|   Microchip Technology Inc.
|   RT-PolarFire IBIS Model
[IBIS ver]   5.0
[File name]   rt-polarfire_hsio_se.ibs
[File Rev]   1.3
[Date]   Thu June 05 2025
[Source] Simulated Models ONLY.
   All data is based on Spice simulation. All performed at Microchip Technology Inc.
[Notes]   This IBIS file is for HSIO single ended standards.
   Please refer to rt-polarfire_hsio_diff.ibs for HSIO differential Standards Configurations,
   and refer to rt-polarfire_gpio_se.ibs and rt-polarfire_gpio_diff.ibs for GPIO Configurations.
   The package parasitics of various package types are given.
   Uncomment the appropriate package before simulations.
   Revision History
   Rev 1.3: 05-Jun-2025
   - Added RLC information for RTPF500ZT-FCG1509 Die-Package combination
   - Added RLC information for RTPF500ZT-CG1509 Die-Package combination
   - Added RLC information for RTPF500ZT-LG1509 Die-Package combination
   - Added RLC information for RTPF500T-LG1509 Die-Package combination
   - This IBIS model file is applicable to all RTPF500T variants
   - RTPF500T/TL/TLS/TS
   - RTPF500ZT/ZTL/ZTLS/ZTS
   Rev 1.2: 22-Nov-2023
   - Added mixed mode receiver support:
   - Input buffers: LVCMOS12_135_ODT-OFF,LVCMOS12_135_ODT-120,LVCMOS12_135_ODT-240,
   HSTL12_18_ODT-OFF,HSTL12_15_ODT-OFF,HSTL12_135_ODT-OFF,
   HSTL135_18_ODT-OFF,HSTL135_15_ODT-OFF,HSTL15_18_ODT-OFF,
   HSUL12_18_ODT-OFF,HSUL12_18_ODT-60,HSUL12_18_ODT-120,HSUL12_18_ODT-240,
   HSUL12_15_ODT-OFF,HSUL12_15_ODT-60,HSUL12_15_ODT-120,HSUL12_15_ODT-240,
   HSUL12_135_ODT-OFF,HSUL12_135_ODT-60,HSUL12_135_ODT-120,HSUL12_135_ODT-240,
   POD12_18_ODT-OFF,POD12_15_ODT-OFF,POD12_135_ODT-OFF,SSTL135_18_ODT-OFF,
   SSTL135_15_ODT-OFF,SSTL15_18_ODT-OFF
   - Updated Pin and Pin Mapping section
   Rev 1.1: 6-Jul-2022
   - Added LPDDR4 LVSTL11 I/O standard
[Disclaimer] This information is for board design considerations.
   Simulation based V/I curves contained in this model file are
   considered preliminary until verified against bench
   measurements. Maximum currents may vary from part to part but
   should not exceed maximum I/V curves provided in this model file.
[Copyright]  (c) 2025, Microchip Technology Inc., All Rights Reserved.
| ADDITIONAL NOTES
| Warnings for ISSO Pullup, Pulldown currents being non-zero maybe ignored.
| The naming conventions used in the signal_name/model_name are as follows:
| SLEW-#  - Slew setting,OFF or ON represented by #
| HYST-#  - Hysteresis setting,OFF or ON represented by #
| #mA   - Driver current strength, value represented by #
| #ohm   - Driver impedance mode, value represented by #
| ODT-#   - Series on-die termination, impedance value represented by #
| C1   - Refers to Class-I driver models
| C2   - Refers to Class-II driver models
| #_I   - Refers to input models ,  model name represented by #
| #_O   - Refers to output models , model name represented by #
| IBIS MODEL CHECKLIST
| Microchip Technology Inc. is dedicated to releasing quality IBIS models to customers.
| The following items have been
| verified for this IBIS model before release:
| 1)  Checked IBIS model by the golden parser ibischk5 [Complete]
| 2)  Ensured no errors reported by golden parser
|   for the IBIS model [Complete]
| 3)  Defined Vinl and Vinh for receivers [Complete]
| 4)  Defined Standard Load and Vmeas values for drivers [Complete]
| 5)  Defined overshoots for drivers and receivers [NA]
| 6)  Validated Ramp Values[]
| 7)  Defined V-T Tables for all output drivers [Complete]
| 8)  Validated [Diff Pins] [NA]
| 9)  Verified Package Parasitics [Complete]
| 10) Defined Standard Load Parameters and Specifications
|   for waveforms [Complete]
| 11) Defined and Validate Pin mappings [Complete]
| 12) Verified C_comp_pullup and C_comp_pulldown Values []
| 13) Visually Inspected I-V Curves and V-T Tables  [Complete]
| 14) Presented Typ/Min/Max Values in the correct order for
|   all tables and parameters [Complete]
| 15) Simulated all output models with standard load and
|   switching through Vmeas [Complete]
| 16) Simulated all receiver models  [Complete]
| 17) Validated Models selectors. [NA]
| 18) Visually inspected Spice and IBIS correlation for
|   a) Typical VT Curves [Complete]
|   b) Minimum VT Curves [Complete]
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[Component]   RTPolarFire
[Manufacturer]   Microchip Technology Inc.
[Package]
|   typ   min   max
|RTPF500T
R_pkg   6.87585   NA   NA   |   RTPF500T-CG1509
L_pkg   14.5627nH   NA   NA   |   RTPF500T-CG1509
C_pkg   5.64467pF   NA   NA   |   RTPF500T-CG1509
|RTPF500T
|R_pkg   6.87585   NA   NA   |   RTPF500T-LG1509
|L_pkg   14.5627nH   NA   NA   |   RTPF500T-LG1509
|C_pkg   5.64467pF   NA   NA   |   RTPF500T-LG1509
|RTPF500ZT
|R_pkg   6.87585   NA   NA   |   RTPF500ZT-CG1509
|L_pkg   14.5627nH   NA   NA   |   RTPF500ZT-CG1509
|C_pkg   5.64467pF   NA   NA   |   RTPF500ZT-CG1509
|RTPF500ZT
|R_pkg   6.87585   NA   NA   |   RTPF500ZT-LG1509
|L_pkg   14.5627nH   NA   NA   |   RTPF500ZT-LG1509
|C_pkg   5.64467pF   NA   NA   |   RTPF500ZT-LG1509
|RTPF500ZT
|R_pkg   1.83029   NA   NA   |   RTPF500ZT-FCG1509
|L_pkg   9.9441nH   NA   NA   |   RTPF500ZT-FCG1509
|C_pkg   3.8557pF   NA   NA   |   RTPF500ZT-FCG1509
| End Header
| The PIN numbers given below are examples. They do not correspond to
| device pin numbers.
[Pin]   signal_name   model_name   R_pin   L_pin   C_pin
1   LVCMOS18_8mA_SLEW-OFF_O   LVCMOS18_8mA_SLEW-OFF_HSIO_O
2   LVCMOS18_2mA_SLEW-OFF_O   LVCMOS18_2mA_SLEW-OFF_HSIO_O
3   LVCMOS18_4mA_SLEW-OFF_O   LVCMOS18_4mA_SLEW-OFF_HSIO_O
4   LVCMOS18_6mA_SLEW-OFF_O   LVCMOS18_6mA_SLEW-OFF_HSIO_O
5   LVCMOS18_10mA_SLEW-OFF_O   LVCMOS18_10mA_SLEW-OFF_HSIO_O
6   LVCMOS18_12mA_SLEW-OFF_O   LVCMOS18_12mA_SLEW-OFF_HSIO_O
7   LVCMOS15_8mA_SLEW-OFF_O   LVCMOS15_8mA_SLEW-OFF_HSIO_O
8   LVCMOS15_2mA_SLEW-OFF_O   LVCMOS15_2mA_SLEW-OFF_HSIO_O
9   LVCMOS15_4mA_SLEW-OFF_O   LVCMOS15_4mA_SLEW-OFF_HSIO_O
10   LVCMOS15_6mA_SLEW-OFF_O   LVCMOS15_6mA_SLEW-OFF_HSIO_O
11   LVCMOS15_10mA_SLEW-OFF_O   LVCMOS15_10mA_SLEW-OFF_HSIO_O
12   LVCMOS12_8mA_SLEW-OFF_O   LVCMOS12_8mA_SLEW-OFF_HSIO_O
13   LVCMOS12_2mA_SLEW-OFF_O   LVCMOS12_2mA_SLEW-OFF_HSIO_O
14   LVCMOS12_4mA_SLEW-OFF_O   LVCMOS12_4mA_SLEW-OFF_HSIO_O
15   LVCMOS12_6mA_SLEW-OFF_O   LVCMOS12_6mA_SLEW-OFF_HSIO_O
16   LVCMOS12_10mA_SLEW-OFF_O   LVCMOS12_10mA_SLEW-OFF_HSIO_O
17   SSTL18_C1_60ohm_SLEW-OFF_O   SSTL18_C1_60ohm_SLEW-OFF_HSIO_O
18   SSTL18_C1_80ohm_SLEW-OFF_O   SSTL18_C1_80ohm_SLEW-OFF_HSIO_O
19   SSTL18_C1_48ohm_SLEW-OFF_O   SSTL18_C1_48ohm_SLEW-OFF_HSIO_O
20   SSTL18_C1_40ohm_SLEW-OFF_O   SSTL18_C1_40ohm_SLEW-OFF_HSIO_O
21   SSTL18_C2_40ohm_SLEW-OFF_O   SSTL18_C2_40ohm_SLEW-OFF_HSIO_O
22   SSTL18_C2_48ohm_SLEW-OFF_O   SSTL18_C2_48ohm_SLEW-OFF_HSIO_O
23   SSTL18_C2_34ohm_SLEW-OFF_O   SSTL18_C2_34ohm_SLEW-OFF_HSIO_O
24   SSTL18_C2_30ohm_SLEW-OFF_O   SSTL18_C2_30ohm_SLEW-OFF_HSIO_O
25   SSTL15_C1_40ohm_SLEW-OFF_O   SSTL15_C1_40ohm_SLEW-OFF_HSIO_O
26   SSTL15_C1_48ohm_SLEW-OFF_O   SSTL15_C1_48ohm_SLEW-OFF_HSIO_O
27   SSTL15_C2_34ohm_SLEW-OFF_O   SSTL15_C2_34ohm_SLEW-OFF_HSIO_O
28   SSTL15_C2_30ohm_SLEW-OFF_O   SSTL15_C2_30ohm_SLEW-OFF_HSIO_O
29   SSTL15_C2_27ohm_SLEW-OFF_O   SSTL15_C2_27ohm_SLEW-OFF_HSIO_O
30   SSTL135_C1_40ohm_SLEW-OFF_O   SSTL135_C1_40ohm_SLEW-OFF_HSIO_O
31   SSTL135_C1_48ohm_SLEW-OFF_O   SSTL135_C1_48ohm_SLEW-OFF_HSIO_O
32   SSTL135_C2_34ohm_SLEW-OFF_O   SSTL135_C2_34ohm_SLEW-OFF_HSIO_O
33   SSTL135_C2_30ohm_SLEW-OFF_O   SSTL135_C2_30ohm_SLEW-OFF_HSIO_O
34   SSTL135_C2_27ohm_SLEW-OFF_O   SSTL135_C2_27ohm_SLEW-OFF_HSIO_O
35   HSUL18_C1_55ohm_SLEW-OFF_O   HSUL18_C1_55ohm_SLEW-OFF_HSIO_O
36   HSUL18_C1_60ohm_SLEW-OFF_O   HSUL18_C1_60ohm_SLEW-OFF_HSIO_O
37   HSUL18_C1_40ohm_SLEW-OFF_O   HSUL18_C1_40ohm_SLEW-OFF_HSIO_O
38   HSUL18_C1_34ohm_SLEW-OFF_O   HSUL18_C1_34ohm_SLEW-OFF_HSIO_O
39   HSUL18_C2_25ohm_SLEW-OFF_O   HSUL18_C2_25ohm_SLEW-OFF_HSIO_O
40   HSUL18_C2_30ohm_SLEW-OFF_O   HSUL18_C2_30ohm_SLEW-OFF_HSIO_O
41   HSUL18_C2_27ohm_SLEW-OFF_O   HSUL18_C2_27ohm_SLEW-OFF_HSIO_O
42   HSUL18_C2_22ohm_SLEW-OFF_O   HSUL18_C2_22ohm_SLEW-OFF_HSIO_O
43   HSTL15_C1_50ohm_SLEW-OFF_O   HSTL15_C1_50ohm_SLEW-OFF_HSIO_O
44   HSTL15_C1_60ohm_SLEW-OFF_O   HSTL15_C1_60ohm_SLEW-OFF_HSIO_O
45   HSTL15_C1_40ohm_SLEW-OFF_O   HSTL15_C1_40ohm_SLEW-OFF_HSIO_O
46   HSTL15_C1_34ohm_SLEW-OFF_O   HSTL15_C1_34ohm_SLEW-OFF_HSIO_O
47   HSTL15_C2_25ohm_SLEW-OFF_O   HSTL15_C2_25ohm_SLEW-OFF_HSIO_O
48   HSTL15_C2_30ohm_SLEW-OFF_O   HSTL15_C2_30ohm_SLEW-OFF_HSIO_O
49   HSTL15_C2_27ohm_SLEW-OFF_O   HSTL15_C2_27ohm_SLEW-OFF_HSIO_O
50   HSTL15_C2_22ohm_SLEW-OFF_O   HSTL15_C2_22ohm_SLEW-OFF_HSIO_O
51   HSTL135_C1_50ohm_SLEW-OFF_O   HSTL135_C1_50ohm_SLEW-OFF_HSIO_O
52   HSTL135_C1_60ohm_SLEW-OFF_O   HSTL135_C1_60ohm_SLEW-OFF_HSIO_O
53   HSTL135_C1_40ohm_SLEW-OFF_O   HSTL135_C1_40ohm_SLEW-OFF_HSIO_O
54   HSTL135_C1_34ohm_SLEW-OFF_O   HSTL135_C1_34ohm_SLEW-OFF_HSIO_O
55   HSTL135_C2_25ohm_SLEW-OFF_O   HSTL135_C2_25ohm_SLEW-OFF_HSIO_O
56   HSTL135_C2_30ohm_SLEW-OFF_O   HSTL135_C2_30ohm_SLEW-OFF_HSIO_O
57   HSTL135_C2_27ohm_SLEW-OFF_O   HSTL135_C2_27ohm_SLEW-OFF_HSIO_O
58   HSTL135_C2_22ohm_SLEW-OFF_O   HSTL135_C2_22ohm_SLEW-OFF_HSIO_O
59   HSUL12_40ohm_SLEW-OFF_O   HSUL12_40ohm_SLEW-OFF_HSIO_O
60   HSUL12_120ohm_SLEW-OFF_O   HSUL12_120ohm_SLEW-OFF_HSIO_O
61   HSUL12_80ohm_SLEW-OFF_O   HSUL12_80ohm_SLEW-OFF_HSIO_O
62   HSUL12_60ohm_SLEW-OFF_O   HSUL12_60ohm_SLEW-OFF_HSIO_O
63   HSUL12_48ohm_SLEW-OFF_O   HSUL12_48ohm_SLEW-OFF_HSIO_O
64   HSUL12_34ohm_SLEW-OFF_O   HSUL12_34ohm_SLEW-OFF_HSIO_O
65   POD12_C1_48ohm_SLEW-OFF_O   POD12_C1_48ohm_SLEW-OFF_HSIO_O
66   POD12_C1_60ohm_SLEW-OFF_O   POD12_C1_60ohm_SLEW-OFF_HSIO_O
67   POD12_C1_40ohm_SLEW-OFF_O   POD12_C1_40ohm_SLEW-OFF_HSIO_O
68   POD12_C2_34ohm_SLEW-OFF_O   POD12_C2_34ohm_SLEW-OFF_HSIO_O
69   POD12_C2_30ohm_SLEW-OFF_O   POD12_C2_30ohm_SLEW-OFF_HSIO_O
70   POD12_C2_27ohm_SLEW-OFF_O   POD12_C2_27ohm_SLEW-OFF_HSIO_O
71   HSTL12_C1_50ohm_SLEW-OFF_O   HSTL12_C1_50ohm_SLEW-OFF_HSIO_O
72   HSTL12_C2_25ohm_SLEW-OFF_O   HSTL12_C2_25ohm_SLEW-OFF_HSIO_O
73   LVCMOS18_ODT-OFF_HYST-ON_I   LVCMOS18_ODT-OFF_HYST-ON_HSIO_I
74   LVCMOS18_ODT-OFF_HYST-OFF_I   LVCMOS18_ODT-OFF_HYST-OFF_HSIO_I
75   LVCMOS18_ODT-120_HYST-ON_I   LVCMOS18_ODT-120_HYST-ON_HSIO_I
76   LVCMOS18_ODT-240_HYST-ON_I   LVCMOS18_ODT-240_HYST-ON_HSIO_I
77   LVCMOS18_ODT-120_HYST-OFF_I   LVCMOS18_ODT-120_HYST-OFF_HSIO_I
78   LVCMOS18_ODT-240_HYST-OFF_I   LVCMOS18_ODT-240_HYST-OFF_HSIO_I
79   LVCMOS15_18_ODT-OFF_HYST-ON_I   LVCMOS15_18_ODT-OFF_HYST-ON_HSIO_I
80   LVCMOS15_18_ODT-OFF_HYST-OFF_I   LVCMOS15_18_ODT-OFF_HYST-OFF_HSIO_I
81   LVCMOS15_18_ODT-120_HYST-ON_I   LVCMOS15_18_ODT-120_HYST-ON_HSIO_I
82   LVCMOS15_18_ODT-240_HYST-ON_I   LVCMOS15_18_ODT-240_HYST-ON_HSIO_I
83   LVCMOS15_18_ODT-120_HYST-OFF_I   LVCMOS15_18_ODT-120_HYST-OFF_HSIO_I
84   LVCMOS15_18_ODT-240_HYST-OFF_I   LVCMOS15_18_ODT-240_HYST-OFF_HSIO_I
85   LVCMOS15_ODT-OFF_HYST-ON_I   LVCMOS15_ODT-OFF_HYST-ON_HSIO_I
86   LVCMOS15_ODT-OFF_HYST-OFF_I   LVCMOS15_ODT-OFF_HYST-OFF_HSIO_I
87   LVCMOS15_ODT-120_HYST-ON_I   LVCMOS15_ODT-120_HYST-ON_HSIO_I
88   LVCMOS15_ODT-240_HYST-ON_I   LVCMOS15_ODT-240_HYST-ON_HSIO_I
89   LVCMOS15_ODT-120_HYST-OFF_I   LVCMOS15_ODT-120_HYST-OFF_HSIO_I
90   LVCMOS15_ODT-240_HYST-OFF_I   LVCMOS15_ODT-240_HYST-OFF_HSIO_I
91   LVCMOS12_18_ODT-OFF_HYST-OFF_I   LVCMOS12_18_ODT-OFF_HYST-OFF_HSIO_I
92   LVCMOS12_15_ODT-OFF_HYST-OFF_I   LVCMOS12_15_ODT-OFF_HYST-OFF_HSIO_I
93   LVCMOS12_18_ODT-120_HYST-OFF_I   LVCMOS12_18_ODT-120_HYST-OFF_HSIO_I
94   LVCMOS12_15_ODT-120_HYST-OFF_I   LVCMOS12_15_ODT-120_HYST-OFF_HSIO_I
95   LVCMOS12_18_ODT-240_HYST-OFF_I   LVCMOS12_18_ODT-240_HYST-OFF_HSIO_I
96   LVCMOS12_15_ODT-240_HYST-OFF_I   LVCMOS12_15_ODT-240_HYST-OFF_HSIO_I
97   LVCMOS12_ODT-OFF_HYST-OFF_I   LVCMOS12_ODT-OFF_HYST-OFF_HSIO_I
98   LVCMOS12_ODT-120_HYST-OFF_I   LVCMOS12_ODT-120_HYST-OFF_HSIO_I
99   LVCMOS12_ODT-240_HYST-OFF_I   LVCMOS12_ODT-240_HYST-OFF_HSIO_I
100   SSTL18_ODT-OFF_HYST-OFF_I   SSTL18_ODT-OFF_HYST-OFF_HSIO_I
101   SSTL18_ODT-50_HYST-OFF_I   SSTL18_ODT-50_HYST-OFF_HSIO_I
102   SSTL18_ODT-150_HYST-OFF_I   SSTL18_ODT-150_HYST-OFF_HSIO_I
103   SSTL18_ODT-75_HYST-OFF_I   SSTL18_ODT-75_HYST-OFF_HSIO_I
104   SSTL15_ODT-OFF_HYST-OFF_I   SSTL15_ODT-OFF_HYST-OFF_HSIO_I
105   SSTL15_ODT-60_HYST-OFF_I   SSTL15_ODT-60_HYST-OFF_HSIO_I
106   SSTL15_ODT-120_HYST-OFF_I   SSTL15_ODT-120_HYST-OFF_HSIO_I
107   SSTL15_ODT-40_HYST-OFF_I   SSTL15_ODT-40_HYST-OFF_HSIO_I
108   SSTL15_ODT-30_HYST-OFF_I   SSTL15_ODT-30_HYST-OFF_HSIO_I
109   SSTL15_ODT-20_HYST-OFF_I   SSTL15_ODT-20_HYST-OFF_HSIO_I
110   SSTL135_ODT-OFF_HYST-OFF_I   SSTL135_ODT-OFF_HYST-OFF_HSIO_I
111   SSTL135_ODT-60_HYST-OFF_I   SSTL135_ODT-60_HYST-OFF_HSIO_I
112   SSTL135_ODT-120_HYST-OFF_I   SSTL135_ODT-120_HYST-OFF_HSIO_I
113   SSTL135_ODT-40_HYST-OFF_I   SSTL135_ODT-40_HYST-OFF_HSIO_I
114   SSTL135_ODT-30_HYST-OFF_I   SSTL135_ODT-30_HYST-OFF_HSIO_I
115   SSTL135_ODT-20_HYST-OFF_I   SSTL135_ODT-20_HYST-OFF_HSIO_I
116   HSUL18_ODT-OFF_HYST-OFF_I   HSUL18_ODT-OFF_HYST-OFF_HSIO_I
117   HSUL18_ODT-50_HYST-OFF_I   HSUL18_ODT-50_HYST-OFF_HSIO_I
118   HSTL15_ODT-OFF_HYST-OFF_I   HSTL15_ODT-OFF_HYST-OFF_HSIO_I
119   HSTL15_ODT-50_HYST-OFF_I   HSTL15_ODT-50_HYST-OFF_HSIO_I
120   HSTL135_ODT-OFF_HYST-OFF_I   HSTL135_ODT-OFF_HYST-OFF_HSIO_I
121   HSTL135_ODT-50_HYST-OFF_I   HSTL135_ODT-50_HYST-OFF_HSIO_I
122   HSUL12_ODT-OFF_HYST-OFF_I   HSUL12_ODT-OFF_HYST-OFF_HSIO_I
123   HSUL12_ODT-60_HYST-OFF_I   HSUL12_ODT-60_HYST-OFF_HSIO_I
124   HSUL12_ODT-240_HYST-OFF_I   HSUL12_ODT-240_HYST-OFF_HSIO_I
125   HSUL12_ODT-120_HYST-OFF_I   HSUL12_ODT-120_HYST-OFF_HSIO_I
126   POD12_ODT-OFF_HYST-OFF_I   POD12_ODT-OFF_HYST-OFF_HSIO_I
127   POD12_ODT-60_HYST-OFF_I   POD12_ODT-60_HYST-OFF_HSIO_I
128   POD12_ODT-240_HYST-OFF_I   POD12_ODT-240_HYST-OFF_HSIO_I
129   POD12_ODT-120_HYST-OFF_I   POD12_ODT-120_HYST-OFF_HSIO_I
130   POD12_ODT-80_HYST-OFF_I   POD12_ODT-80_HYST-OFF_HSIO_I
131   POD12_ODT-48_HYST-OFF_I   POD12_ODT-48_HYST-OFF_HSIO_I
132   POD12_ODT-40_HYST-OFF_I   POD12_ODT-40_HYST-OFF_HSIO_I
133   POD12_ODT-34_HYST-OFF_I   POD12_ODT-34_HYST-OFF_HSIO_I
134   HSTL12_ODT-OFF_HYST-OFF_I   HSTL12_ODT-OFF_HYST-OFF_HSIO_I
135   HSTL12_ODT-50_HYST-OFF_I   HSTL12_ODT-50_HYST-OFF_HSIO_I
136   LVSTL11_C1_40ohm_SLEW-OFF_O   LVSTL11_C1_40ohm_SLEW-OFF_HSIO_O
137   LVSTL11_C1_120ohm_SLEW-OFF_O   LVSTL11_C1_120ohm_SLEW-OFF_HSIO_O
138   LVSTL11_C1_80ohm_SLEW-OFF_O   LVSTL11_C1_80ohm_SLEW-OFF_HSIO_O
139   LVSTL11_C1_60ohm_SLEW-OFF_O   LVSTL11_C1_60ohm_SLEW-OFF_HSIO_O
140   LVSTL11_C1_48ohm_SLEW-OFF_O   LVSTL11_C1_48ohm_SLEW-OFF_HSIO_O
141   LVSTL11_C1_34ohm_SLEW-OFF_O   LVSTL11_C1_34ohm_SLEW-OFF_HSIO_O
142   LVSTL11_ODT-OFF_HYST-OFF_I   LVSTL11_ODT-OFF_HYST-OFF_HSIO_I
143   LVSTL11_ODT-60_HYST-OFF_I   LVSTL11_ODT-60_HYST-OFF_HSIO_I
144   LVSTL11_ODT-120_HYST-OFF_I   LVSTL11_ODT-120_HYST-OFF_HSIO_I
145   LVSTL11_ODT-80_HYST-OFF_I   LVSTL11_ODT-80_HYST-OFF_HSIO_I
146   LVSTL11_ODT-48_HYST-OFF_I   LVSTL11_ODT-48_HYST-OFF_HSIO_I
147   LVSTL11_ODT-40_HYST-OFF_I   LVSTL11_ODT-40_HYST-OFF_HSIO_I
148   LVCMOS12_135_ODT-OFF_HYST-OFF_I   LVCMOS12_135_ODT-OFF_HYST-OFF_HSIO_I
149   LVCMOS12_135_ODT-120_HYST-OFF_I   LVCMOS12_135_ODT-120_HYST-OFF_HSIO_I
150   LVCMOS12_135_ODT-240_HYST-OFF_I   LVCMOS12_135_ODT-240_HYST-OFF_HSIO_I
151   HSTL12_18_ODT-OFF_HYST-OFF_I   HSTL12_18_ODT-OFF_HYST-OFF_HSIO_I
152   HSTL12_15_ODT-OFF_HYST-OFF_I   HSTL12_15_ODT-OFF_HYST-OFF_HSIO_I
153   HSTL12_135_ODT-OFF_HYST-OFF_I   HSTL12_135_ODT-OFF_HYST-OFF_HSIO_I
154   HSTL135_18_ODT-OFF_HYST-OFF_I   HSTL135_18_ODT-OFF_HYST-OFF_HSIO_I
155   HSTL135_15_ODT-OFF_HYST-OFF_I   HSTL135_15_ODT-OFF_HYST-OFF_HSIO_I
156   HSTL15_18_ODT-OFF_HYST-OFF_I   HSTL15_18_ODT-OFF_HYST-OFF_HSIO_I
157   HSUL12_18_ODT-OFF_HYST-OFF_I   HSUL12_18_ODT-OFF_HYST-OFF_HSIO_I
158   HSUL12_15_ODT-OFF_HYST-OFF_I   HSUL12_15_ODT-OFF_HYST-OFF_HSIO_I
159   HSUL12_135_ODT-OFF_HYST-OFF_I   HSUL12_135_ODT-OFF_HYST-OFF_HSIO_I
160   HSUL12_18_ODT-60_HYST-OFF_I   HSUL12_18_ODT-60_HYST-OFF_HSIO_I
161   HSUL12_15_ODT-60_HYST-OFF_I   HSUL12_15_ODT-60_HYST-OFF_HSIO_I
162   HSUL12_135_ODT-60_HYST-OFF_I   HSUL12_135_ODT-60_HYST-OFF_HSIO_I
163   HSUL12_18_ODT-240_HYST-OFF_I   HSUL12_18_ODT-240_HYST-OFF_HSIO_I
164   HSUL12_15_ODT-240_HYST-OFF_I   HSUL12_15_ODT-240_HYST-OFF_HSIO_I
165   HSUL12_135_ODT-240_HYST-OFF_I   HSUL12_135_ODT-240_HYST-OFF_HSIO_I
166   HSUL12_18_ODT-120_HYST-OFF_I   HSUL12_18_ODT-120_HYST-OFF_HSIO_I
167   HSUL12_15_ODT-120_HYST-OFF_I   HSUL12_15_ODT-120_HYST-OFF_HSIO_I
168   HSUL12_135_ODT-120_HYST-OFF_I   HSUL12_135_ODT-120_HYST-OFF_HSIO_I
169   POD12_18_ODT-OFF_HYST-OFF_I   POD12_18_ODT-OFF_HYST-OFF_HSIO_I
170   POD12_15_ODT-OFF_HYST-OFF_I   POD12_15_ODT-OFF_HYST-OFF_HSIO_I
171   POD12_135_ODT-OFF_HYST-OFF_I   POD12_135_ODT-OFF_HYST-OFF_HSIO_I
172   SSTL135_18_ODT-OFF_HYST-OFF_I   SSTL135_18_ODT-OFF_HYST-OFF_HSIO_I
173   SSTL135_15_ODT-OFF_HYST-OFF_I   SSTL135_15_ODT-OFF_HYST-OFF_HSIO_I
174   SSTL15_18_ODT-OFF_HYST-OFF_I   SSTL15_18_ODT-OFF_HYST-OFF_HSIO_I
175   VDDI   POWER
176   VSS   GND
[Pin Mapping]   pulldown_ref   pullup_ref   gnd_clamp_ref   power_clamp_ref   ext_ref
1   VSS   VDDI   VSS   VDDI
2   VSS   VDDI   VSS   VDDI
3   VSS   VDDI   VSS   VDDI
4   VSS   VDDI   VSS   VDDI
5   VSS   VDDI   VSS   VDDI
6   VSS   VDDI   VSS   VDDI
7   VSS   VDDI   VSS   VDDI
8   VSS   VDDI   VSS   VDDI
9   VSS   VDDI   VSS   VDDI
10   VSS   VDDI   VSS   VDDI
11   VSS   VDDI   VSS   VDDI
12   VSS   VDDI   VSS   VDDI
13   VSS   VDDI   VSS   VDDI
14   VSS   VDDI   VSS   VDDI
15   VSS   VDDI   VSS   VDDI
16   VSS   VDDI   VSS   VDDI
17   VSS   VDDI   VSS   VDDI
18   VSS   VDDI   VSS   VDDI
19   VSS   VDDI   VSS   VDDI
20   VSS   VDDI   VSS   VDDI
21   VSS   VDDI   VSS   VDDI
22   VSS   VDDI   VSS   VDDI
23   VSS   VDDI   VSS   VDDI
24   VSS   VDDI   VSS   VDDI
25   VSS   VDDI   VSS   VDDI
26   VSS   VDDI   VSS   VDDI
27   VSS   VDDI   VSS   VDDI
28   VSS   VDDI   VSS   VDDI
29   VSS   VDDI   VSS   VDDI
30   VSS   VDDI   VSS   VDDI
31   VSS   VDDI   VSS   VDDI
32   VSS   VDDI   VSS   VDDI
33   VSS   VDDI   VSS   VDDI
34   VSS   VDDI   VSS   VDDI
35   VSS   VDDI   VSS   VDDI
36   VSS   VDDI   VSS   VDDI
37   VSS   VDDI   VSS   VDDI
38   VSS   VDDI   VSS   VDDI
39   VSS   VDDI   VSS   VDDI
40   VSS   VDDI   VSS   VDDI
41   VSS   VDDI   VSS   VDDI
42   VSS   VDDI   VSS   VDDI
43   VSS   VDDI   VSS   VDDI
44   VSS   VDDI   VSS   VDDI
45   VSS   VDDI   VSS   VDDI
46   VSS   VDDI   VSS   VDDI
47   VSS   VDDI   VSS   VDDI
48   VSS   VDDI   VSS   VDDI
49   VSS   VDDI   VSS   VDDI
50   VSS   VDDI   VSS   VDDI
51   VSS   VDDI   VSS   VDDI
52   VSS   VDDI   VSS   VDDI
53   VSS   VDDI   VSS   VDDI
54   VSS   VDDI   VSS   VDDI
55   VSS   VDDI   VSS   VDDI
56   VSS   VDDI   VSS   VDDI
57   VSS   VDDI   VSS   VDDI
58   VSS   VDDI   VSS   VDDI
59   VSS   VDDI   VSS   VDDI
60   VSS   VDDI   VSS   VDDI
61   VSS   VDDI   VSS   VDDI
62   VSS   VDDI   VSS   VDDI
63   VSS   VDDI   VSS   VDDI
64   VSS   VDDI   VSS   VDDI
65   VSS   VDDI   VSS   VDDI
66   VSS   VDDI   VSS   VDDI
67   VSS   VDDI   VSS   VDDI
68   VSS   VDDI   VSS   VDDI
69   VSS   VDDI   VSS   VDDI
70   VSS   VDDI   VSS   VDDI
71   VSS   VDDI   VSS   VDDI
72   VSS   VDDI   VSS   VDDI
73   VSS   VDDI   VSS   VDDI
74   VSS   VDDI   VSS   VDDI
75   VSS   VDDI   VSS   VDDI
76   VSS   VDDI   VSS   VDDI
77   VSS   VDDI   VSS   VDDI
78   VSS   VDDI   VSS   VDDI
79   VSS   VDDI   VSS   VDDI
80   VSS   VDDI   VSS   VDDI
81   VSS   VDDI   VSS   VDDI
82   VSS   VDDI   VSS   VDDI
83   VSS   VDDI   VSS   VDDI
84   VSS   VDDI   VSS   VDDI
85   VSS   VDDI   VSS   VDDI
86   VSS   VDDI   VSS   VDDI
87   VSS   VDDI   VSS   VDDI
88   VSS   VDDI   VSS   VDDI
89   VSS   VDDI   VSS   VDDI
90   VSS   VDDI   VSS   VDDI
91   VSS   VDDI   VSS   VDDI
92   VSS   VDDI   VSS   VDDI
93   VSS   VDDI   VSS   VDDI
94   VSS   VDDI   VSS   VDDI
95   VSS   VDDI   VSS   VDDI
96   VSS   VDDI   VSS   VDDI
97   VSS   VDDI   VSS   VDDI
98   VSS   VDDI   VSS   VDDI
99   VSS   VDDI   VSS   VDDI
100   VSS   VDDI   VSS   VDDI
101   VSS   VDDI   VSS   VDDI
102   VSS   VDDI   VSS   VDDI
103   VSS   VDDI   VSS   VDDI
104   VSS   VDDI   VSS   VDDI
105   VSS   VDDI   VSS   VDDI
106   VSS   VDDI   VSS   VDDI
107   VSS   VDDI   VSS   VDDI
108   VSS   VDDI   VSS   VDDI
109   VSS   VDDI   VSS   VDDI
110   VSS   VDDI   VSS   VDDI
111   VSS   VDDI   VSS   VDDI
112   VSS   VDDI   VSS   VDDI
113   VSS   VDDI   VSS   VDDI
114   VSS   VDDI   VSS   VDDI
115   VSS   VDDI   VSS   VDDI
116   VSS   VDDI   VSS   VDDI
117   VSS   VDDI   VSS   VDDI
118   VSS   VDDI   VSS   VDDI
119   VSS   VDDI   VSS   VDDI
120   VSS   VDDI   VSS   VDDI
121   VSS   VDDI   VSS   VDDI
122   VSS   VDDI   VSS   VDDI
123   VSS   VDDI   VSS   VDDI
124   VSS   VDDI   VSS   VDDI
125   VSS   VDDI   VSS   VDDI
126   VSS   VDDI   VSS   VDDI
127   VSS   VDDI   VSS   VDDI
128   VSS   VDDI   VSS   VDDI
129   VSS   VDDI   VSS   VDDI
130   VSS   VDDI   VSS   VDDI
131   VSS   VDDI   VSS   VDDI
132   VSS   VDDI   VSS   VDDI
133   VSS   VDDI   VSS   VDDI
134   VSS   VDDI   VSS   VDDI
135   VSS   VDDI   VSS   VDDI
136   VSS   VDDI   VSS   VDDI
137   VSS   VDDI   VSS   VDDI
138   VSS   VDDI   VSS   VDDI
139   VSS   VDDI   VSS   VDDI
140   VSS   VDDI   VSS   VDDI
141   VSS   VDDI   VSS   VDDI
142   VSS   VDDI   VSS   VDDI
143   VSS   VDDI   VSS   VDDI
144   VSS   VDDI   VSS   VDDI
145   VSS   VDDI   VSS   VDDI
146   VSS   VDDI   VSS   VDDI
147   VSS   VDDI   VSS   VDDI
148   VSS   VDDI   VSS   VDDI
149   VSS   VDDI   VSS   VDDI
150   VSS   VDDI   VSS   VDDI
151   VSS   VDDI   VSS   VDDI
152   VSS   VDDI   VSS   VDDI
153   VSS   VDDI   VSS   VDDI
154   VSS   VDDI   VSS   VDDI
155   VSS   VDDI   VSS   VDDI
156   VSS   VDDI   VSS   VDDI
157   VSS   VDDI   VSS   VDDI
158   VSS   VDDI   VSS   VDDI
159   VSS   VDDI   VSS   VDDI
160   VSS   VDDI   VSS   VDDI
161   VSS   VDDI   VSS   VDDI
162   VSS   VDDI   VSS   VDDI
163   VSS   VDDI   VSS   VDDI
164   VSS   VDDI   VSS   VDDI
165   VSS   VDDI   VSS   VDDI
166   VSS   VDDI   VSS   VDDI
167   VSS   VDDI   VSS   VDDI
168   VSS   VDDI   VSS   VDDI
169   VSS   VDDI   VSS   VDDI
170   VSS   VDDI   VSS   VDDI
171   VSS   VDDI   VSS   VDDI
172   VSS   VDDI   VSS   VDDI
173   VSS   VDDI   VSS   VDDI
174   VSS   VDDI   VSS   VDDI
175   NC   VDDI
176   VSS   NC
| Models and submodels in the file (174): LVCMOS18_8mA_SLEW-OFF_HSIO_O (Output), LVCMOS18_2mA_SLEW-OFF_HSIO_O (Output), LVCMOS18_4mA_SLEW-OFF_HSIO_O (Output), LVCMOS18_6mA_SLEW-OFF_HSIO_O (Output), LVCMOS18_10mA_SLEW-OFF_HSIO_O (Output), LVCMOS18_12mA_SLEW-OFF_HSIO_O (Output), LVCMOS15_8mA_SLEW-OFF_HSIO_O (Output), LVCMOS15_2mA_SLEW-OFF_HSIO_O (Output), LVCMOS15_4mA_SLEW-OFF_HSIO_O (Output), LVCMOS15_6mA_SLEW-OFF_HSIO_O (Output), LVCMOS15_10mA_SLEW-OFF_HSIO_O (Output), LVCMOS12_8mA_SLEW-OFF_HSIO_O (Output), LVCMOS12_2mA_SLEW-OFF_HSIO_O (Output), LVCMOS12_4mA_SLEW-OFF_HSIO_O (Output), LVCMOS12_6mA_SLEW-OFF_HSIO_O (Output), LVCMOS12_10mA_SLEW-OFF_HSIO_O (Output), SSTL18_C1_60ohm_SLEW-OFF_HSIO_O (Output), SSTL18_C1_80ohm_SLEW-OFF_HSIO_O (Output), SSTL18_C1_48ohm_SLEW-OFF_HSIO_O (Output), SSTL18_C1_40ohm_SLEW-OFF_HSIO_O (Output), SSTL18_C2_40ohm_SLEW-OFF_HSIO_O (Output), SSTL18_C2_48ohm_SLEW-OFF_HSIO_O (Output), SSTL18_C2_34ohm_SLEW-OFF_HSIO_O (Output), SSTL18_C2_30ohm_SLEW-OFF_HSIO_O (Output), SSTL15_C1_40ohm_SLEW-OFF_HSIO_O (Output), SSTL15_C1_48ohm_SLEW-OFF_HSIO_O (Output), SSTL15_C2_34ohm_SLEW-OFF_HSIO_O (Output), SSTL15_C2_30ohm_SLEW-OFF_HSIO_O (Output), SSTL15_C2_27ohm_SLEW-OFF_HSIO_O (Output), SSTL135_C1_40ohm_SLEW-OFF_HSIO_O (Output), SSTL135_C1_48ohm_SLEW-OFF_HSIO_O (Output), SSTL135_C2_34ohm_SLEW-OFF_HSIO_O (Output), SSTL135_C2_30ohm_SLEW-OFF_HSIO_O (Output), SSTL135_C2_27ohm_SLEW-OFF_HSIO_O (Output), HSUL18_C1_55ohm_SLEW-OFF_HSIO_O (Output), HSUL18_C1_60ohm_SLEW-OFF_HSIO_O (Output), HSUL18_C1_40ohm_SLEW-OFF_HSIO_O (Output), HSUL18_C1_34ohm_SLEW-OFF_HSIO_O (Output), HSUL18_C2_25ohm_SLEW-OFF_HSIO_O (Output), HSUL18_C2_30ohm_SLEW-OFF_HSIO_O (Output), HSUL18_C2_27ohm_SLEW-OFF_HSIO_O (Output), HSUL18_C2_22ohm_SLEW-OFF_HSIO_O (Output), HSTL15_C1_50ohm_SLEW-OFF_HSIO_O (Output), HSTL15_C1_60ohm_SLEW-OFF_HSIO_O (Output), HSTL15_C1_40ohm_SLEW-OFF_HSIO_O (Output), HSTL15_C1_34ohm_SLEW-OFF_HSIO_O (Output), HSTL15_C2_25ohm_SLEW-OFF_HSIO_O (Output), HSTL15_C2_30ohm_SLEW-OFF_HSIO_O (Output), HSTL15_C2_27ohm_SLEW-OFF_HSIO_O (Output), HSTL15_C2_22ohm_SLEW-OFF_HSIO_O (Output), HSTL135_C1_50ohm_SLEW-OFF_HSIO_O (Output), HSTL135_C1_60ohm_SLEW-OFF_HSIO_O (Output), HSTL135_C1_40ohm_SLEW-OFF_HSIO_O (Output), HSTL135_C1_34ohm_SLEW-OFF_HSIO_O (Output), HSTL135_C2_25ohm_SLEW-OFF_HSIO_O (Output), HSTL135_C2_30ohm_SLEW-OFF_HSIO_O (Output), HSTL135_C2_27ohm_SLEW-OFF_HSIO_O (Output), HSTL135_C2_22ohm_SLEW-OFF_HSIO_O (Output), HSUL12_40ohm_SLEW-OFF_HSIO_O (Output), HSUL12_120ohm_SLEW-OFF_HSIO_O (Output), HSUL12_80ohm_SLEW-OFF_HSIO_O (Output), HSUL12_60ohm_SLEW-OFF_HSIO_O (Output), HSUL12_48ohm_SLEW-OFF_HSIO_O (Output), HSUL12_34ohm_SLEW-OFF_HSIO_O (Output), POD12_C1_48ohm_SLEW-OFF_HSIO_O (Output), POD12_C1_60ohm_SLEW-OFF_HSIO_O (Output), POD12_C1_40ohm_SLEW-OFF_HSIO_O (Output), POD12_C2_34ohm_SLEW-OFF_HSIO_O (Output), POD12_C2_30ohm_SLEW-OFF_HSIO_O (Output), POD12_C2_27ohm_SLEW-OFF_HSIO_O (Output), HSTL12_C1_50ohm_SLEW-OFF_HSIO_O (Output), HSTL12_C2_25ohm_SLEW-OFF_HSIO_O (Output), LVCMOS18_ODT-OFF_HYST-ON_HSIO_I (Input), LVCMOS18_ODT-OFF_HYST-OFF_HSIO_I (Input), LVCMOS18_ODT-120_HYST-ON_HSIO_I (Input), LVCMOS18_ODT-240_HYST-ON_HSIO_I (Input), LVCMOS18_ODT-120_HYST-OFF_HSIO_I (Input), LVCMOS18_ODT-240_HYST-OFF_HSIO_I (Input), LVCMOS15_18_ODT-OFF_HYST-ON_HSIO_I (Input), LVCMOS15_18_ODT-OFF_HYST-OFF_HSIO_I (Input)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
